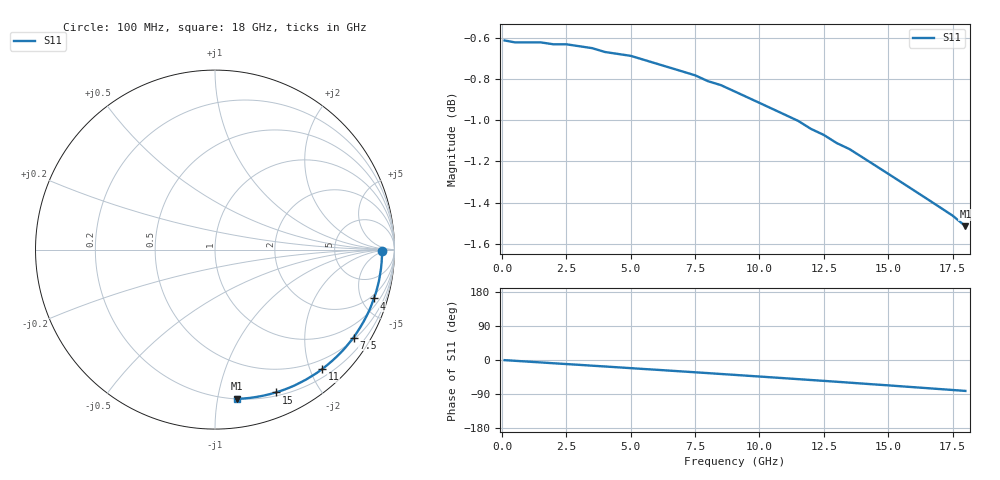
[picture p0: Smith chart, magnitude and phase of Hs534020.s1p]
!HSCH-5320 and HSCH-5340 Schottky diodes
!S-parameters at 20 microamp external bias.  Last upda
# ghz s ma r 50
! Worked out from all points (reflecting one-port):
!   37 points, 100 MHz to 18 GHz, reference 50 ohm
!   lowest |S11| = -1.5 dB at 18 GHz (marker M1), VSWR 11.50, Z = 10.1 - j56.9 ohm
!   phase of S11 starts at -0 deg and turns -81 deg over the sweep
!   S11 on the Smith chart (normalised r, x): 100 MHz: 28, -3; 4 GHz: 1.63, -6.23; 7.5 GHz: 0.56, -3.35; 11 GHz: 0.33, -2.19; 15 GHz: 0.24, -1.49; 18 GHz: 0.20, -1.14
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0.1  0.932 -0.4
1.5  0.931 -6.4
2  0.93 -8.6
2.5  0.93 -10.7
3  0.929 -12.8
3.5  0.928 -15.0
4  0.926 -17.1
5  0.924 -21.5
5.5  0.922 -23.7
6  0.92 -25.8
7  0.916 -30.2
7.5  0.914 -32.4
8.5  0.909 -36.9
9  0.906 -39.1
9.5  0.903 -41.4
10  0.9 -43.6
11  0.894 -48.2
11.5  0.891 -50.5
12.5  0.884 -55.1
13.5  0.877 -59.8
14  0.873 -62.2
14.5  0.869 -64.6
15  0.865 -66.9
15.5  0.861 -69.4
16  0.857 -71.8
17  0.849 -76.7
17.5  0.845 -79.1
18  0.84 -81.6
